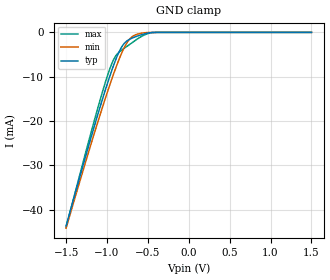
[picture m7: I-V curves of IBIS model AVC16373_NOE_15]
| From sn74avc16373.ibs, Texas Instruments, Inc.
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[Model]   AVC16373_NOE_15
Model_type  Input
Vinl=0.49
Vinh=1.04
| variable   typ   min   max
C_comp   1.72pF   1.30pF   2.07pF
[Temperature Range]   40   100   -40
| Ambient temperature   25   85   -40
[Voltage range]   1.5   1.4   1.6
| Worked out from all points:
|   GND clamp passes 1 mA (typ) near -0.65 V on its own axis
[GND Clamp]
| AVC16373_NOE_15
|   Voltage   I(typ)   I(min)   I(max)
-1.5V     -43.63mA   -44.14mA   -44.02mA
-1.16V    -21.5mA    -23.06mA   -20.23mA
-1.05V    -14.75mA   -16.59mA   -13.09mA
-970mV    -10.14mA   -12.09mA   -8.455mA
-900mV    -6.492mA   -8.396mA   -5.515mA
-825mV    -3.443mA   -4.871mA   -4.055mA
-755mV    -1.92mA    -2.322mA   -3.132mA
-695mV    -1.309mA   -1.025mA   -2.358mA
-635mV    -878.3uA   -443.8uA   -1.573mA
-550mV    -385.2uA   -118.7uA   -652.1uA
-430mV    -20.2uA    -12.29uA   -29.52uA
1.5V      196.2pA    665.6pA    8.947pA
